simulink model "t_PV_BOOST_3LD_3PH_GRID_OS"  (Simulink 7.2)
settings: Solver=ode3  StartTime=0.0  StopTime=0.2  FixedStep=10e-6  MaxStep=1e-5  RelTol=1e-5  AbsTol=1e-5
PreLoadFcn:
  | INIT_PWM_Con
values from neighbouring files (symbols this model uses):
  I_B = INP    [INIT_PWM_Con.m]    (also in INIT_B6_2L_3Ph_IGBT_OS.m = INS; INIT_B6_3L_3Ph_IGBT_OS.m = INS; INIT_PWM_2L.m; INIT_PWM_3L.m)
  UNP = ULLP/sqrt(3)    [INIT_PWM_Con.m]    (also in INIT_B6_2L_3Ph_IGBT_OS.m; INIT_B6_3L_3Ph_IGBT_OS.m; INIT_PWM_2L.m; INIT_PWM_3L.m)
  VDC = 1200    [INIT_PWM_Con.m]    (also in INIT_B6_2L_3Ph_IGBT_OS.m = 600; INIT_B6_3L_3Ph_IGBT_OS.m = 1000; INIT_PWM_2L.m = 600; INIT_PWM_3L.m)

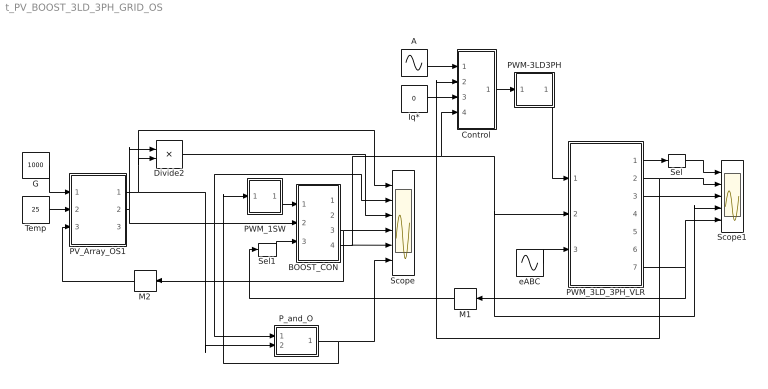
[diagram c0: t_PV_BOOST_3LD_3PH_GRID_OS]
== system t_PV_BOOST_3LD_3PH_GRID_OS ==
  A : Sin  Amplitude=.9  Frequency=2*pi*50  Phase="[0  -2*pi/3  -4*pi/3 ]"  SampleTime=0
  BOOST_CON : Subsystem  mask{L1=5e-3, IL0=100, C1=5e-3, UC0=1200, R1=1e5}
      mask prompts: L1 "Inductance L1"; IL0 "Initial Current"; C1 "Capacitance"; UC0 "Initial Voltage"; R1 "Load Resistance"
      mask help: Open Source boost Converter Input Vector u: u[0]= T1.gate u[1]= E.v u[2]= IDC.i Output Vector y: y[0]= T1.I y[1]= D1.I y[2]= L1.I y[3]= C1.V Parameter Vector p: p[0]= L1.L p[1]= L1.iL0 p[2]= C1.C p[3]= C1.vC0 p[4]= R1.r You can pause the simulation during running, change the Parameters you want and continue the Simulation
  Control : Subsystem
  Divide2 : Product  Inputs=**
  G : Constant  Value=1000  OutDataType=sfix(16)  OutScaling=2^0
  Iq* : Constant  Value=0  OutDataType=sfix(16)  OutScaling=2^0
  M1 : Memory  Orientation=left
  M2 : Memory  Orientation=left
  PV_Array_OS1 : Subsystem  mask{Isc0=5.28, Ud0=44.5, Ki=2e-3, Kv=-0.1558, n=1.0, RS=0.7, RP=400, NC=72, NMs=20, NMp=15, C=1e-4, vC0=0, RL=10000}
      mask prompts: Isc0 "Short Circuit Current at STC Isc0/Module"; Ud0 "Open Circuit Voltage at STC Ud0/Module"; Ki "Short Circuit Current Temp Coeff. Ki/Module"; Kv "Open Circuit Voltage Temp. Coeff. Kv/Module"; n "Diode Idealty Factor n"; RS "Series Resistance Rs"; RP "Parallel Resistance RP"; NC "Number Cells"; NMs "Number Series Modules"; NMp "Number Parallel Modules"; C "Load Capacitor"; vC0 "init Cap Voltage"; RL "Load Res."
      mask help: PV_Array_OS with parameters: N_Cells/Module (NC), N_Series connected Module (NMs) and N_parallel connected Module (NMp) Input Vector u: u[0]=G u[1]=T u[2]=ILd Output Vector y: y[0]=PV.I y[1]=PV.V y[2]=C.I Parameter Vector p: p[0]=Isc0 p[1]=Ud0 p[2]=Ki p[3]=Kv p[4]=n p[5]=RS p[6]=RP p[7]=NC p[8]=NMs p[9]=NMp p[10]=C p[11]=vC0 p[12]=RL You can pause the simulation during running, change the Parameters you want and continue the Simulation
  PWM-3LD3PH : Subsystem  mask(PWM-3LD3PH){FT=500, PHT=0, A=0.5, O1=0.5, O2=-0.5, DT=1e-6}
      mask prompts: FT "Frequency of Trian Sig."; PHT "Phase Angle of Trian. Sig."; A "Amplitude of Trian. Sig."; O1 "Offset of 1st Trian"; O2 "Offset of 2nd Trian."; DT "Dead Time"
      mask help: Pulse Width Modulation for 3 Phase 3 Level Neutral point clamped Converter
  PWM_1SW : Subsystem  mask(PWMtr){FS=1e3}
      mask prompts: FS "Frequency"
  PWM_3LD_3PH_VLR : Subsystem  mask(pwm_3LD_3PH_VLR_OS){RL=1e-3, LL=10e-3}
      mask prompts: RL "Load Resistance"; LL "Load Inductance"
      mask help: Open Source 3-Level NPC PWM_3PH Converter with VLR load Input Vector u: u{0:11}= gating Signals u[12]/2= VDC1, VDC2 u{13:15}= EA,EB,EC Output Vector y: y{0:2}= Va,Vb,Vc y{3:5}= Ia,Ib,Ic y[6]= Vab.V y{7:9} = T1.I,D1.I,T1.V y{10:12}= T2.I,D2.I,T2.V y[13]= D5.I y[14]= D5.V y[15]= IDC1 y[16]= IDC2 Parameter Vector p: p[0]=RL p[1]=LL You can pause the simulation during running, change the Parameters you want and continue the Simulation
  P_and_O : Subsystem  mask{DeltaD=0.0001}
      mask help: MPPT controller based on the Perturb & Observe algorithm. D output = Duty cycle of the boost converter (value between 0 and 1) DeltaD = 0.0001; Increment value used to increase/decrease the duty cycle D
  Scope : Scope  NumInputPorts=6
  Scope1 : Scope  NumInputPorts=5
  Sel : Selector  InputPortWidth=3  IndexOptions=Index vector (dialog)  Indices=[1 ]  OutputSizes=1
  Sel1 : Selector  InputPortWidth=2  IndexOptions=Index vector (dialog)  Indices=[1 ]  OutputSizes=1
  Temp : Constant  Value=25  OutDataType=sfix(16)  OutScaling=2^0
  eABC : Sin  Amplitude=UNP  Frequency=2*pi*50  Phase="[0  -2*pi/3  -4*pi/3 ]"  SampleTime=0
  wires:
  PWM_1SW/1(Out1) -> BOOST_CON/1(sw)
  P_and_O/1(D) -> PWM_1SW/1(In1), Scope/6
  PV_Array_OS1/2(PV_V) -> BOOST_CON/2(E), P_and_O/1(V), Scope/2, Divide2/1
  BOOST_CON/3(iL) -> Scope/4, M2/1
  PV_Array_OS1/1(PV_I) -> P_and_O/2(I), Divide2/2, Scope/1
  BOOST_CON/4(vC) -> Scope/5, PWM_3LD_3PH_VLR/2(vDC), Scope1/4, Control/4(UDC)
  G/1 -> PV_Array_OS1/1(G)
  Temp/1 -> PV_Array_OS1/2(Temp)
  PWM-3LD3PH/1(Out1) -> PWM_3LD_3PH_VLR/1(Sw)
  eABC/1 -> PWM_3LD_3PH_VLR/3(E_ABC)
  PWM_3LD_3PH_VLR/1(vABC) -> Sel/1
  PWM_3LD_3PH_VLR/2(iABC) -> Scope1/2, Control/2(Iwr)
  PWM_3LD_3PH_VLR/3(vAB) -> Scope1/3
  Sel/1 -> Scope1/1
  PWM_3LD_3PH_VLR/7(iDC1,iDC2) -> M1/1, Scope1/5
  M1/1 -> Sel1/1
  M2/1 -> PV_Array_OS1/3(ILd)
  A/1 -> Control/1(UNP)
  Control/1(A) -> PWM-3LD3PH/1(In1)
  Iq*/1 -> Control/3(Iq*)
  Divide2/1 -> Scope/3
  Sel1/1 -> BOOST_CON/3(IDC)

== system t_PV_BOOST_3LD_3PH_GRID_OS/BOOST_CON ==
  sw : Inport  OutDataType=sfix(16)  OutScaling=2^0
  E : Inport  Port=2  OutDataType=sfix(16)  OutScaling=2^0
  IDC : Inport  Port=3  OutDataType=sfix(16)  OutScaling=2^0
  BOOST : S-Function  FunctionName=s_boost_OS  Parameters="[L1  IL0  C1   UC0  R1]"  EnableBusSupport=off
  Mux1 : Mux  Inputs=3
  iT : Outport  OutDataType=sfix(16)  OutScaling=2^0
  iD : Outport  Port=2  OutDataType=sfix(16)  OutScaling=2^0
  iL : Outport  Port=3  OutDataType=sfix(16)  OutScaling=2^0
  vC : Outport  Port=4  OutDataType=sfix(16)  OutScaling=2^0
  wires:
  IDC/1 -> Mux1/3
  BOOST/4 -> vC/1
  BOOST/3 -> iL/1
  BOOST/2 -> iD/1
  BOOST/1 -> iT/1
  E/1 -> Mux1/2
  sw/1 -> Mux1/1
  Mux1/1 -> BOOST/1

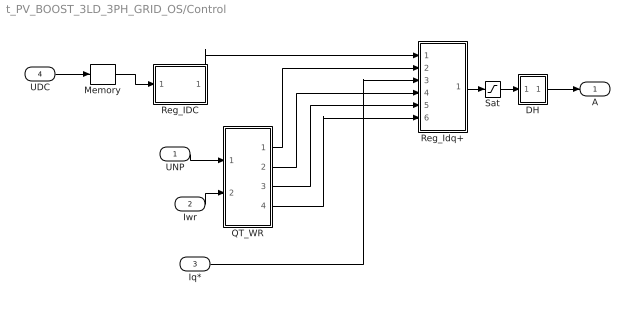
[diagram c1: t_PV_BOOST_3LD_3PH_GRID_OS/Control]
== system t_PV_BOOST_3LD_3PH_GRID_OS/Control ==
  UNP : Inport
  Iwr : Inport  Port=2
  Iq* : Inport  Port=3
  UDC : Inport  Port=4
  DH : Subsystem
  Memory : Memory
  QT_WR : Subsystem
  Reg_IDC : Subsystem
  Reg_Idq+ : Subsystem
  Sat : Saturate  UpperLimit=1  LowerLimit=-1
  A : Outport
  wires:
  QT_WR/4(Ud) -> Reg_Idq+/6(Ud)
  QT_WR/1(Id1) -> Reg_Idq+/2(Id1)
  QT_WR/2(Iq1) -> Reg_Idq+/4(Iq1)
  Iq*/1 -> Reg_Idq+/3(Iq1*)
  QT_WR/3(th1) -> Reg_Idq+/5(th)
  Iwr/1 -> QT_WR/2(I_WR)
  UNP/1 -> QT_WR/1(UNP)
  DH/1(O) -> A/1
  Reg_Idq+/1(A+) -> Sat/1
  Sat/1 -> DH/1(I)
  UDC/1 -> Memory/1
  Memory/1 -> Reg_IDC/1(UDC)
  Reg_IDC/1(Id1*) -> Reg_Idq+/1(Id1*)

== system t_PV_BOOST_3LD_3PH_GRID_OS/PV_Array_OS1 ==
  G : Inport
  Temp : Inport  Port=2
  ILd : Inport  Port=3
  Mux : Mux  Inputs=3
  t_PV_Array_OS : S-Function  FunctionName=s_PV_Array_OS  Parameters="[Isc0  Ud0  Ki  Kv  n    RS  RP NC  NMs NMp C  vC0  RL]"  EnableBusSupport=off
  PV_I : Outport
  PV_V : Outport  Port=2
  C_I : Outport  Port=3
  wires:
  Mux/1 -> t_PV_Array_OS/1
  G/1 -> Mux/1
  Temp/1 -> Mux/2
  ILd/1 -> Mux/3
  t_PV_Array_OS/1 -> PV_I/1
  t_PV_Array_OS/2 -> PV_V/1
  t_PV_Array_OS/3 -> C_I/1

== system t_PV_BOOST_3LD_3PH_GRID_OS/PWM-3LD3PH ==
  In1 : Inport  OutDataType=sfix(16)  OutScaling=2^0
  Demux1 : Demux  Outputs=3
  Mux1 : Mux  Inputs=3
  PWM-3LD1PH : Subsystem  mask(PWM-3LD_1PH){FT=FT, PHT=PHT, A=A, O1=O1, O2=O2, DT=DT}
      mask prompts: FT "Frequency of Trian Sig."; PHT "Phase Angle of Trian. Sig."; A "Amplitude of Trian. Sig."; O1 "Offset of 1st Trian"; O2 "Offset of 2nd Trian."; DT "Dead Time"
      mask help: Pulse Width Modulation for 1 Leg of 3 Level Neutral point clamped Converter
  PWM-3LD1PH1 : Subsystem  mask(PWM-3LD_1PH){FT=FT, PHT=PHT, A=A, O1=O1, O2=O2, DT=DT}
      mask prompts: FT "Frequency of Trian Sig."; PHT "Phase Angle of Trian. Sig."; A "Amplitude of Trian. Sig."; O1 "Offset of 1st Trian"; O2 "Offset of 2nd Trian."; DT "Dead Time"
      mask help: Pulse Width Modulation for 1 Leg of 3 Level Neutral point clamped Converter
  PWM-3LD1PH2 : Subsystem  mask(PWM-3LD_1PH){FT=FT, PHT=PHT, A=A, O1=O1, O2=O2, DT=DT}
      mask prompts: FT "Frequency of Trian Sig."; PHT "Phase Angle of Trian. Sig."; A "Amplitude of Trian. Sig."; O1 "Offset of 1st Trian"; O2 "Offset of 2nd Trian."; DT "Dead Time"
      mask help: Pulse Width Modulation for 1 Leg of 3 Level Neutral point clamped Converter
  Out1 : Outport
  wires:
  In1/1 -> Demux1/1
  Demux1/3 -> PWM-3LD1PH2/1(In1)
  Demux1/2 -> PWM-3LD1PH1/1(In1)
  Demux1/1 -> PWM-3LD1PH/1(In1)
  Mux1/1 -> Out1/1
  PWM-3LD1PH2/1(Out1) -> Mux1/3
  PWM-3LD1PH1/1(Out1) -> Mux1/2
  PWM-3LD1PH/1(Out1) -> Mux1/1

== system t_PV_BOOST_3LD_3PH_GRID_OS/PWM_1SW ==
  In1 : Inport  OutDataType=sfix(16)  OutScaling=2^0
  Relay : Relay  OutDataType=sfix(16)  OutScaling=2^0
  SoToG : Subsystem  mask(SoToG){T=1/FS}
      mask prompts: T "Period Time"
  Sum : Sum  Inputs=+-  OutDataType=sfix(16)  OutScaling=2^0
  Out1 : Outport  InitialOutput=0
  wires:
  Relay/1 -> Out1/1
  SoToG/1(O) -> Sum/2
  In1/1 -> Sum/1
  Sum/1 -> Relay/1

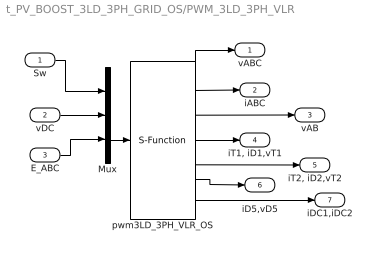
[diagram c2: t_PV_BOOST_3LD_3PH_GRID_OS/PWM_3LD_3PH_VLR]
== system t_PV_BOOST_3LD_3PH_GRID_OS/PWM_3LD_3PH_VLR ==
  Sw : Inport  OutDataType=sfix(16)  OutScaling=2^0
  vDC : Inport  Port=2  OutDataType=sfix(16)  OutScaling=2^0
  E_ABC : Inport  Port=3  OutDataType=sfix(16)  OutScaling=2^0
  Mux : Mux  Inputs="[12 1  3]"
  pwm3LD_3PH_VLR_OS : S-Function  FunctionName=s_pwm_3LD_3PH_VLR_OS  Parameters="[RL  LL]"  EnableBusSupport=off
  vABC : Outport  OutDataType=sfix(16)  OutScaling=2^0
  iABC : Outport  Port=2  OutDataType=sfix(16)  OutScaling=2^0
  vAB : Outport  Port=3  OutDataType=sfix(16)  OutScaling=2^0
  "iT1, iD1,vT1" : Outport  Port=4  OutDataType=sfix(16)  OutScaling=2^0
  "iT2, iD2,vT2" : Outport  Port=5  OutDataType=sfix(16)  OutScaling=2^0
  iD5,vD5 : Outport  Port=6  OutDataType=sfix(16)  OutScaling=2^0
  iDC1,iDC2 : Outport  Port=7  OutDataType=sfix(16)  OutScaling=2^0
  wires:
  Sw/1 -> Mux/1
  vDC/1 -> Mux/2
  Mux/1 -> pwm3LD_3PH_VLR_OS/1
  E_ABC/1 -> Mux/3
  pwm3LD_3PH_VLR_OS/1 -> vABC/1
  pwm3LD_3PH_VLR_OS/4 -> "iT1, iD1,vT1"/1
  pwm3LD_3PH_VLR_OS/2 -> iABC/1
  pwm3LD_3PH_VLR_OS/3 -> vAB/1
  pwm3LD_3PH_VLR_OS/5 -> "iT2, iD2,vT2"/1
  pwm3LD_3PH_VLR_OS/6 -> iD5,vD5/1
  pwm3LD_3PH_VLR_OS/7 -> iDC1,iDC2/1

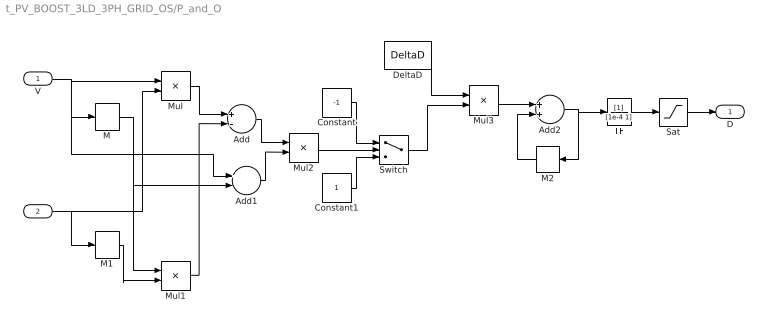
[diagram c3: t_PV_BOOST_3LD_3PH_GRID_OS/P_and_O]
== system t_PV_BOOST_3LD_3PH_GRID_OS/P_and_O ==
  V : Inport  OutDataType=sfix(16)  OutScaling=2^0
  I : Inport  Port=2  OutDataType=sfix(16)  OutScaling=2^0
  Add : Sum  Inputs=+-  OutDataType=sfix(16)  OutScaling=2^-10
  Add1 : Sum  Inputs=+-  OutDataType=sfix(16)  OutScaling=2^-10
  Add2 : Sum  OutDataType=sfix(16)  OutScaling=2^-10
  Constant : Constant  Value=-1  OutDataType=sfix(16)  OutScaling=2^0
  Constant1 : Constant  OutDataType=sfix(16)  OutScaling=2^0
  DeltaD : Constant  Value=DeltaD  OutDataType=sfix(16)  OutScaling=2^0
  M : Memory
  M1 : Memory
  M2 : Memory  Orientation=left
  Mul{,1..3} (4 alike) : Product  Inputs=**  OutDataType=sfix(16)  OutScaling=2^-10
  Sat : Saturate  UpperLimit=1  LowerLimit=0  OutDataType=sfix(16)  OutScaling=2^0
  Switch : Switch  OutDataType=sfix(16)  OutScaling=2^0
  TF : TransferFcn  Denominator=[1e-4 1]
  D : Outport  OutDataType=sfix(16)  OutScaling=2^0
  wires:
  Sat/1 -> D/1
  TF/1 -> Sat/1
  M2/1 -> Add2/2
  Add2/1 -> TF/1, M2/1
  Mul3/1 -> Add2/1
  DeltaD/1 -> Mul3/1
  Switch/1 -> Mul3/2
  Constant1/1 -> Switch/3
  Constant/1 -> Switch/1
  Mul2/1 -> Switch/2
  Add1/1 -> Mul2/2
  Add/1 -> Mul2/1
  Mul1/1 -> Add/2
  Mul/1 -> Add/1
  M1/1 -> Mul1/2
  M/1 -> Add1/2, Mul1/1
  V/1 -> Add1/1, M/1, Mul/1
  I/1 -> M1/1, Mul/2

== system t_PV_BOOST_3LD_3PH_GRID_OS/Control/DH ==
  I : Inport
  Gain : Gain  Gain=0.5
  MinMax : MinMax
  MinMax1 : MinMax  Function=max
  Sum6 : Sum  Inputs=--
  Sum7 : Sum
  O : Outport  InitialOutput=0
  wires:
  Sum7/1 -> O/1
  Gain/1 -> Sum7/2
  Sum6/1 -> Gain/1
  MinMax1/1 -> Sum6/2
  MinMax/1 -> Sum6/1
  I/1 -> Sum7/1, MinMax/1, MinMax1/1

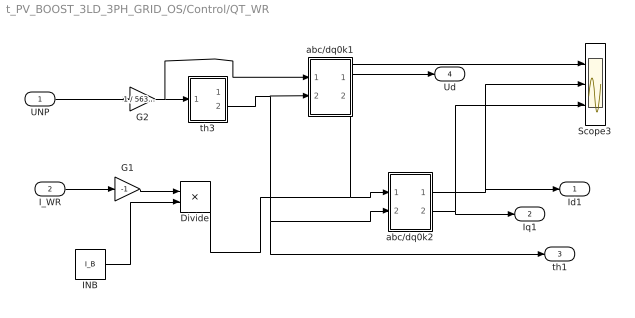
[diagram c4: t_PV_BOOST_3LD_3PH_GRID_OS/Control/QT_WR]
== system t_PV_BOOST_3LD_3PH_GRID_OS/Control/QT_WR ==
  UNP : Inport
  I_WR : Inport  Port=2
  Divide : Product  Inputs=*/  OutDataType=sfix(16)  OutScaling=2^-10
  G1 : Gain  Gain=-1
  G2 : Gain  Gain=1 / 563.39
  INB : Constant  Value=I_B  OutDataType=sfix(16)  OutScaling=2^0
  Scope3 : Scope  NumInputPorts=3
  abc/dq0k1 : Subsystem
  abc/dq0k2 : Subsystem
  th3 : Subsystem
  Id1 : Outport
  Iq1 : Outport  Port=2
  th1 : Outport  Port=3
  Ud : Outport  Port=4
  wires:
  INB/1 -> Divide/2
  G1/1 -> Divide/1
  Divide/1 -> Scope3/1, abc/dq0k2/1(a)
  UNP/1 -> G2/1
  abc/dq0k1/1(dk) -> Ud/1
  abc/dq0k2/2(qk) -> Scope3/3, Iq1/1
  abc/dq0k2/1(dk) -> Scope3/2, Id1/1
  G2/1 -> abc/dq0k1/1(a), th3/1(abc)
  I_WR/1 -> G1/1
  th3/2(th) -> abc/dq0k2/2(th), th1/1, abc/dq0k1/2(th)

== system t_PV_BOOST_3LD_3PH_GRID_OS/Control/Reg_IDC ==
  UDC : Inport
  Add : Sum
  G4 : Gain  Gain=1/VDC
  PIC1 : Subsystem  mask(PI-controller){Kp=20, Ki=10, Kd=0, lim=10, Ts=-10}
      mask prompts: Kp "Proportional gain (Kp)"; Ki "Integral gain (Ki)"; Kd "Diff. gain (Kd)"; lim "Output limit"; Ts "Sampling time (s)"
      mask help: Proportional-Integral Controller
  Sat : Saturate  UpperLimit=2  LowerLimit=-2
  UC_Reg : Scope  NumInputPorts=3
  UDC* : Constant  Value=1.0
  Id1* : Outport
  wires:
  UDC/1 -> G4/1
  UDC*/1 -> PIC1/1(c*)
  G4/1 -> PIC1/2(c), UC_Reg/3
  PIC1/1(e*) -> UC_Reg/2, Add/2
  Add/1 -> Sat/1
  Sat/1 -> Id1*/1, UC_Reg/1

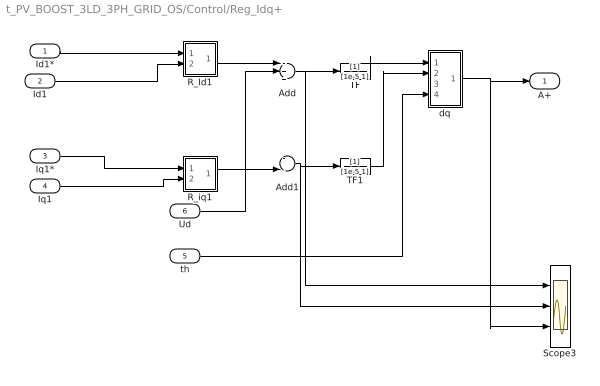
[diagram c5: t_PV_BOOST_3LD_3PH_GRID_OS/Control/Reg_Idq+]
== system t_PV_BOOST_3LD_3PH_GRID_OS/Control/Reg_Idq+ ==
  Id1* : Inport
  Id1 : Inport  Port=2
  Iq1* : Inport  Port=3
  Iq1 : Inport  Port=4
  th : Inport  Port=5
  Ud : Inport  Port=6
  Add : Sum  Inputs=-++
  Add1 : Sum  Inputs=--
  R_Id1 : Subsystem  mask(PI-controller){Kp=1, Ki=100, lim=2, Ts=-1}
      mask prompts: Kp "Proportional gain (Kp)"; Ki "Integral gain (Ki)"; lim "Output limit"; Ts "Sampling time (s)"
      mask help: Proportional-Integral Controller
  R_iq1 : Subsystem  mask(PI-controller){Kp=1, Ki=100, lim=2, Ts=-2}
      mask prompts: Kp "Proportional gain (Kp)"; Ki "Integral gain (Ki)"; lim "Output limit"; Ts "Sampling time (s)"
      mask help: Proportional-Integral Controller
  Scope3 : Scope  NumInputPorts=3
  TF : TransferFcn  Denominator=[1e-5 1]
  TF1 : TransferFcn  Denominator=[1e-5 1]
  dq : Subsystem
  A+ : Outport
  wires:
  Ud/1 -> Add/2
  TF1/1 -> dq/2(qk)
  TF/1 -> dq/1(dk)
  Add1/1 -> Scope3/2, TF1/1
  Add/1 -> Scope3/1, TF/1
  R_iq1/1(e*) -> Add1/2
  R_Id1/1(e*) -> Add/1
  th/1 -> dq/4(th)
  dq/1(a) -> Scope3/3, A+/1
  Id1*/1 -> R_Id1/1(c*)
  Id1/1 -> R_Id1/2(c)
  Iq1*/1 -> R_iq1/1(c*)
  Iq1/1 -> R_iq1/2(c)

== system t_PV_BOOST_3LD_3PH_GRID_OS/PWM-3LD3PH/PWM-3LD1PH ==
  In1 : Inport  OutDataType=sfix(16)  OutScaling=2^0
  Mux : Mux
  SS : Subsystem
  SS1 : Subsystem
  Out1 : Outport
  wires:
  In1/1 -> SS1/1(I1), SS/1(I1)
  SS1/1(O1) -> Mux/2
  SS/2(O2) -> Mux/3
  Mux/1 -> Out1/1
  SS/1(O1) -> Mux/1
  SS1/2(O2) -> Mux/4

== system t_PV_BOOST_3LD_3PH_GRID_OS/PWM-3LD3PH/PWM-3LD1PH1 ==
  In1 : Inport  OutDataType=sfix(16)  OutScaling=2^0
  Mux : Mux
  SS : Subsystem
  SS1 : Subsystem
  Out1 : Outport
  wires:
  SS1/2(O2) -> Mux/4
  SS/1(O1) -> Mux/1
  Mux/1 -> Out1/1
  SS/2(O2) -> Mux/3
  SS1/1(O1) -> Mux/2
  In1/1 -> SS/1(I1), SS1/1(I1)

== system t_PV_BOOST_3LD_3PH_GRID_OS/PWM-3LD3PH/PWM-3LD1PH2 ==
  In1 : Inport  OutDataType=sfix(16)  OutScaling=2^0
  Mux : Mux
  SS : Subsystem
  SS1 : Subsystem
  Out1 : Outport
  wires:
  In1/1 -> SS1/1(I1), SS/1(I1)
  SS1/1(O1) -> Mux/2
  SS/2(O2) -> Mux/3
  Mux/1 -> Out1/1
  SS/1(O1) -> Mux/1
  SS1/2(O2) -> Mux/4

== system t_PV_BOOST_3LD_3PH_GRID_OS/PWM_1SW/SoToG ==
  Clock : Clock
  P : Product  OutDataType=sfix(16)  OutScaling=2^0
  T1 : Constant  Value=T  OutDataType=sfix(16)  OutScaling=2^0
  T2 : Constant  Value=1/T  OutDataType=sfix(16)  OutScaling=2^0
  mod : Math  Operator=mod
  O : Outport
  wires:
  P/1 -> O/1
  mod/1 -> P/1
  T2/1 -> P/2
  T1/1 -> mod/2
  Clock/1 -> mod/1

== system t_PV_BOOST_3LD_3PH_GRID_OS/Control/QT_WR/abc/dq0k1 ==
  a : Inport
  th : Inport  Port=2
  Demux : Demux  Outputs=3
  Fcn : Fcn  Expr=u(1)*cos(u(3)) + u(2)*sin(u(3))
  Fcn1 : Fcn  Expr=-u(1)*sin(u(3)) + u(2)*cos(u(3))
  K : Gain  Gain="2/3*[1   -.5   -.5;  0   sqrt(3)/2   -sqrt(3)/2;  .5    .5    .5]"  Multiplication=Matrix(K*u)
  Mux1 : Mux  Inputs=3
  dk : Outport
  qk : Outport  Port=2
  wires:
  K/1 -> Demux/1
  a/1 -> K/1
  Mux1/1 -> Fcn1/1, Fcn/1
  Fcn/1 -> dk/1
  Fcn1/1 -> qk/1
  th/1 -> Mux1/3
  Demux/1 -> Mux1/1
  Demux/2 -> Mux1/2

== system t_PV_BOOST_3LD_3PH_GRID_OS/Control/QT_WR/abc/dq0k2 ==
  a : Inport
  th : Inport  Port=2
  Demux : Demux  Outputs=3
  Fcn : Fcn  Expr=u(1)*cos(u(3)) + u(2)*sin(u(3))
  Fcn1 : Fcn  Expr=-u(1)*sin(u(3)) + u(2)*cos(u(3))
  K : Gain  Gain="2/3*[1   -.5   -.5;  0   sqrt(3)/2   -sqrt(3)/2;  .5    .5    .5]"  Multiplication=Matrix(K*u)
  Mux1 : Mux  Inputs=3
  dk : Outport
  qk : Outport  Port=2
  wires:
  Demux/2 -> Mux1/2
  Demux/1 -> Mux1/1
  th/1 -> Mux1/3
  Fcn1/1 -> qk/1
  Fcn/1 -> dk/1
  Mux1/1 -> Fcn/1, Fcn1/1
  a/1 -> K/1
  K/1 -> Demux/1

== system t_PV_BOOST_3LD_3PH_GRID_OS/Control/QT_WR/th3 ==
  abc : Inport
  C : ComplexToMagnitudeAngle
  Demux : Demux  Outputs=3
  K : Gain  Gain="2/3*[1   -.5   -.5;  0   sqrt(3)/2   -sqrt(3)/2;  .5    .5    .5]"  Multiplication=Matrix(K*u)
  R : RealImagToComplex
  |u| : Outport
  th : Outport  Port=2
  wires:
  C/1 -> |u|/1
  K/1 -> Demux/1
  abc/1 -> K/1
  Demux/1 -> R/1
  Demux/2 -> R/2
  R/1 -> C/1
  C/2 -> th/1

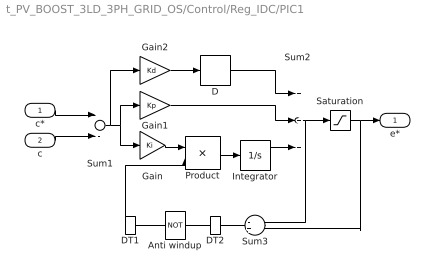
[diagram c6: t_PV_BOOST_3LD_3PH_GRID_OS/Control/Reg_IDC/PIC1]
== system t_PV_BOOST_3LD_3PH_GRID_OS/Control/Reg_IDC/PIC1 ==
  c* : Inport
  c : Inport  Port=2
  Anti windup : Logic  Operator=NOT
  D : Derivative
  DT1 : DataTypeConversion
  DT2 : DataTypeConversion
  Gain : Gain  Gain=Ki
  Gain1 : Gain  Gain=Kp
  Gain2 : Gain  Gain=Kd
  Integrator : Integrator  UpperSaturationLimit=lim  LowerSaturationLimit=-lim
  Product : Product
  Saturation : Saturate  UpperLimit=lim  LowerLimit=-lim
  Sum1 : Sum  Inputs=+-
  Sum2 : Sum  Inputs=+++
  Sum3 : Sum  Inputs=-+
  e* : Outport  InitialOutput=0
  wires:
  Sum3/1 -> DT2/1
  DT2/1 -> Anti windup/1
  Product/1 -> Integrator/1
  Gain/1 -> Product/1
  DT1/1 -> Product/2
  Anti windup/1 -> DT1/1
  Gain1/1 -> Sum2/2
  Sum1/1 -> Gain/1, Gain1/1, Gain2/1
  Sum2/1 -> Sum3/1, Saturation/1
  Saturation/1 -> Sum3/2, e*/1
  c/1 -> Sum1/2
  c*/1 -> Sum1/1
  Integrator/1 -> Sum2/3
  Gain2/1 -> D/1
  D/1 -> Sum2/1

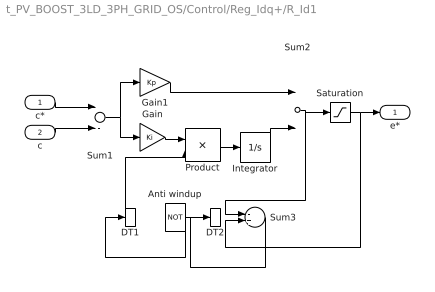
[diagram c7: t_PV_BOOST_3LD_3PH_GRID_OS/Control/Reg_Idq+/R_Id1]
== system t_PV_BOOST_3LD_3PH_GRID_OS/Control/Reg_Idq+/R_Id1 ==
  c* : Inport
  c : Inport  Port=2
  Anti windup : Logic  Operator=NOT
  DT1 : DataTypeConversion
  DT2 : DataTypeConversion
  Gain : Gain  Gain=Ki
  Gain1 : Gain  Gain=Kp
  Integrator : Integrator  UpperSaturationLimit=lim  LowerSaturationLimit=-lim
  Product : Product
  Saturation : Saturate  UpperLimit=lim  LowerLimit=-lim
  Sum1 : Sum  Inputs=+-
  Sum2 : Sum
  Sum3 : Sum  Inputs=-+
  e* : Outport  InitialOutput=0
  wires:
  Sum3/1 -> DT2/1
  DT2/1 -> Anti windup/1
  Product/1 -> Integrator/1
  Gain/1 -> Product/1
  DT1/1 -> Product/2
  Anti windup/1 -> DT1/1
  Gain1/1 -> Sum2/1
  Sum1/1 -> Gain/1, Gain1/1
  Sum2/1 -> Sum3/1, Saturation/1
  Saturation/1 -> Sum3/2, e*/1
  c/1 -> Sum1/2
  c*/1 -> Sum1/1
  Integrator/1 -> Sum2/2

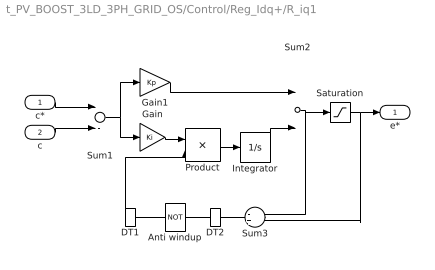
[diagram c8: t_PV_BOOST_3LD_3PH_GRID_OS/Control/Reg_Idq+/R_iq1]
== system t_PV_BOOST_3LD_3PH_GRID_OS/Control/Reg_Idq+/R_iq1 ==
  c* : Inport
  c : Inport  Port=2
  Anti windup : Logic  Operator=NOT
  DT1 : DataTypeConversion
  DT2 : DataTypeConversion
  Gain : Gain  Gain=Ki
  Gain1 : Gain  Gain=Kp
  Integrator : Integrator  UpperSaturationLimit=lim  LowerSaturationLimit=-lim
  Product : Product
  Saturation : Saturate  UpperLimit=lim  LowerLimit=-lim
  Sum1 : Sum  Inputs=+-
  Sum2 : Sum
  Sum3 : Sum  Inputs=-+
  e* : Outport  InitialOutput=0
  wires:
  Integrator/1 -> Sum2/2
  c*/1 -> Sum1/1
  c/1 -> Sum1/2
  Saturation/1 -> e*/1, Sum3/2
  Sum2/1 -> Saturation/1, Sum3/1
  Sum1/1 -> Gain1/1, Gain/1
  Gain1/1 -> Sum2/1
  Anti windup/1 -> DT1/1
  DT1/1 -> Product/2
  Gain/1 -> Product/1
  Product/1 -> Integrator/1
  DT2/1 -> Anti windup/1
  Sum3/1 -> DT2/1

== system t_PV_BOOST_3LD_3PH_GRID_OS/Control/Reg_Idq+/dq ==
  dk : Inport
  qk : Inport  Port=2
  0k : Inport  Port=3
  th : Inport  Port=4
  Fcn : Fcn  Expr=u(1)*cos(u(3)) - u(2)*sin(u(3))
  Fcn1 : Fcn  Expr=u(1)*sin(u(3)) + u(2)*cos(u(3))
  K : Gain  Gain="[1   0  1 ;  -.5   sqrt(3)/2    1 ;  -.5    -sqrt(3)/2    1]"  Multiplication=Matrix(K*u)
  Mux : Mux  Inputs=3
  Mux1 : Mux  Inputs=3
  a : Outport
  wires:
  dk/1 -> Mux/1
  qk/1 -> Mux/2
  Mux/1 -> Fcn/1, Fcn1/1
  K/1 -> a/1
  Mux1/1 -> K/1
  Fcn/1 -> Mux1/1
  Fcn1/1 -> Mux1/2
  th/1 -> Mux/3
  0k/1 -> Mux1/3

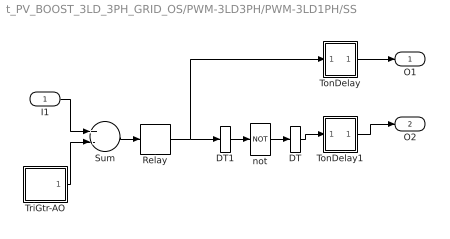
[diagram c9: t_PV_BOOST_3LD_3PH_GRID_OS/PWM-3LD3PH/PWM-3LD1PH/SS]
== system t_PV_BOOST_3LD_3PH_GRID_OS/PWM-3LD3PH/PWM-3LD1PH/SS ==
  I1 : Inport  OutDataType=sfix(16)  OutScaling=2^0
  DT : DataTypeConversion
  DT1 : DataTypeConversion
  Relay : Relay  OutDataType=sfix(16)  OutScaling=2^0
  Sum : Sum  Inputs=+-  OutDataType=sfix(16)  OutScaling=2^0
  TonDelay : Subsystem  mask(TonDelay){DT=DT}
      mask prompts: DT "Dead Time"
      mask help: Turn on dead time to protect against short circuit of the converter leg
  TonDelay1 : Subsystem  mask(TonDelay){DT=DT}
      mask prompts: DT "Dead Time"
      mask help: Turn on dead time to protect against short circuit of the converter leg
  TriGtr-AO : Subsystem  mask(TriGtr-AO){A=A, O=O1, T=1/FT, Td=PHT/FT/180}
      mask prompts: A "Amplitude"; O "Offset"; T "Period Time"; Td "Time Delay"
      mask help: Triangular Wave Generator with variable time delay, variable amplitude and offset
  not : Logic  Operator=NOT  Inputs=1
  O1 : Outport  InitialOutput=0
  O2 : Outport  Port=2  InitialOutput=0
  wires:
  TonDelay/1(s1d) -> O1/1
  Relay/1 -> TonDelay/1(s1), DT1/1
  TonDelay1/1(s1d) -> O2/1
  not/1 -> DT/1
  Sum/1 -> Relay/1
  TriGtr-AO/1(Out1) -> Sum/2
  I1/1 -> Sum/1
  DT/1 -> TonDelay1/1(s1)
  DT1/1 -> not/1

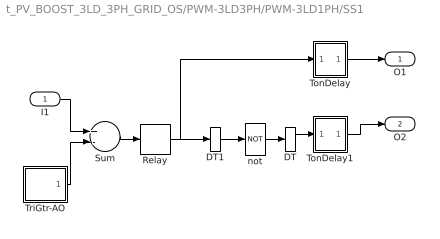
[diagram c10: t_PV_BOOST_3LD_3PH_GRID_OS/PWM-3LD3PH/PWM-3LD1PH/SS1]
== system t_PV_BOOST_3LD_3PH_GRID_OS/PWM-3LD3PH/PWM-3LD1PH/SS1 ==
  I1 : Inport  OutDataType=sfix(16)  OutScaling=2^0
  DT : DataTypeConversion
  DT1 : DataTypeConversion
  Relay : Relay  OutDataType=sfix(16)  OutScaling=2^0
  Sum : Sum  Inputs=+-  OutDataType=sfix(16)  OutScaling=2^0
  TonDelay : Subsystem  mask(TonDelay){DT=DT}
      mask prompts: DT "Dead Time"
      mask help: Turn on dead time to protect against short circuit of the converter leg
  TonDelay1 : Subsystem  mask(TonDelay){DT=DT}
      mask prompts: DT "Dead Time"
      mask help: Turn on dead time to protect against short circuit of the converter leg
  TriGtr-AO : Subsystem  mask(TriGtr-AO){A=A, O=O2, T=1/FT, Td=PHT/FT/180}
      mask prompts: A "Amplitude"; O "Offset"; T "Period Time"; Td "Time Delay"
      mask help: Triangular Wave Generator with variable time delay, variable amplitude and offset
  not : Logic  Operator=NOT  Inputs=1
  O1 : Outport  InitialOutput=0
  O2 : Outport  Port=2  InitialOutput=0
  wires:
  TonDelay/1(s1d) -> O1/1
  Relay/1 -> TonDelay/1(s1), DT1/1
  TonDelay1/1(s1d) -> O2/1
  not/1 -> DT/1
  Sum/1 -> Relay/1
  TriGtr-AO/1(Out1) -> Sum/2
  I1/1 -> Sum/1
  DT/1 -> TonDelay1/1(s1)
  DT1/1 -> not/1

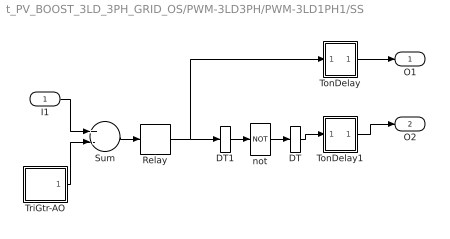
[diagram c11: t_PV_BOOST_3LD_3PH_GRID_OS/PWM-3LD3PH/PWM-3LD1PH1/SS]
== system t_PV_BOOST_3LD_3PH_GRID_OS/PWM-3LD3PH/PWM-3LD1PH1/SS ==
  I1 : Inport  OutDataType=sfix(16)  OutScaling=2^0
  DT : DataTypeConversion
  DT1 : DataTypeConversion
  Relay : Relay  OutDataType=sfix(16)  OutScaling=2^0
  Sum : Sum  Inputs=+-  OutDataType=sfix(16)  OutScaling=2^0
  TonDelay : Subsystem  mask(TonDelay){DT=DT}
      mask prompts: DT "Dead Time"
      mask help: Turn on dead time to protect against short circuit of the converter leg
  TonDelay1 : Subsystem  mask(TonDelay){DT=DT}
      mask prompts: DT "Dead Time"
      mask help: Turn on dead time to protect against short circuit of the converter leg
  TriGtr-AO : Subsystem  mask(TriGtr-AO){A=A, O=O1, T=1/FT, Td=PHT/FT/180}
      mask prompts: A "Amplitude"; O "Offset"; T "Period Time"; Td "Time Delay"
      mask help: Triangular Wave Generator with variable time delay, variable amplitude and offset
  not : Logic  Operator=NOT  Inputs=1
  O1 : Outport  InitialOutput=0
  O2 : Outport  Port=2  InitialOutput=0
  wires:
  DT1/1 -> not/1
  DT/1 -> TonDelay1/1(s1)
  I1/1 -> Sum/1
  TriGtr-AO/1(Out1) -> Sum/2
  Sum/1 -> Relay/1
  not/1 -> DT/1
  TonDelay1/1(s1d) -> O2/1
  Relay/1 -> DT1/1, TonDelay/1(s1)
  TonDelay/1(s1d) -> O1/1

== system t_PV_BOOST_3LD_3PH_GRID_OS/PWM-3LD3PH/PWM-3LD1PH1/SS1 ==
  I1 : Inport  OutDataType=sfix(16)  OutScaling=2^0
  DT : DataTypeConversion
  DT1 : DataTypeConversion
  Relay : Relay  OutDataType=sfix(16)  OutScaling=2^0
  Sum : Sum  Inputs=+-  OutDataType=sfix(16)  OutScaling=2^0
  TonDelay : Subsystem  mask(TonDelay){DT=DT}
      mask prompts: DT "Dead Time"
      mask help: Turn on dead time to protect against short circuit of the converter leg
  TonDelay1 : Subsystem  mask(TonDelay){DT=DT}
      mask prompts: DT "Dead Time"
      mask help: Turn on dead time to protect against short circuit of the converter leg
  TriGtr-AO : Subsystem  mask(TriGtr-AO){A=A, O=O2, T=1/FT, Td=PHT/FT/180}
      mask prompts: A "Amplitude"; O "Offset"; T "Period Time"; Td "Time Delay"
      mask help: Triangular Wave Generator with variable time delay, variable amplitude and offset
  not : Logic  Operator=NOT  Inputs=1
  O1 : Outport  InitialOutput=0
  O2 : Outport  Port=2  InitialOutput=0
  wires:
  DT1/1 -> not/1
  DT/1 -> TonDelay1/1(s1)
  I1/1 -> Sum/1
  TriGtr-AO/1(Out1) -> Sum/2
  Sum/1 -> Relay/1
  not/1 -> DT/1
  TonDelay1/1(s1d) -> O2/1
  Relay/1 -> DT1/1, TonDelay/1(s1)
  TonDelay/1(s1d) -> O1/1

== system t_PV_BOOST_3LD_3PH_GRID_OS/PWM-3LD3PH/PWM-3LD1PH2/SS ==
  I1 : Inport  OutDataType=sfix(16)  OutScaling=2^0
  DT : DataTypeConversion
  DT1 : DataTypeConversion
  Relay : Relay  OutDataType=sfix(16)  OutScaling=2^0
  Sum : Sum  Inputs=+-  OutDataType=sfix(16)  OutScaling=2^0
  TonDelay : Subsystem  mask(TonDelay){DT=DT}
      mask prompts: DT "Dead Time"
      mask help: Turn on dead time to protect against short circuit of the converter leg
  TonDelay1 : Subsystem  mask(TonDelay){DT=DT}
      mask prompts: DT "Dead Time"
      mask help: Turn on dead time to protect against short circuit of the converter leg
  TriGtr-AO : Subsystem  mask(TriGtr-AO){A=A, O=O1, T=1/FT, Td=PHT/FT/180}
      mask prompts: A "Amplitude"; O "Offset"; T "Period Time"; Td "Time Delay"
      mask help: Triangular Wave Generator with variable time delay, variable amplitude and offset
  not : Logic  Operator=NOT  Inputs=1
  O1 : Outport  InitialOutput=0
  O2 : Outport  Port=2  InitialOutput=0
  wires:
  TonDelay/1(s1d) -> O1/1
  Relay/1 -> TonDelay/1(s1), DT1/1
  TonDelay1/1(s1d) -> O2/1
  not/1 -> DT/1
  Sum/1 -> Relay/1
  TriGtr-AO/1(Out1) -> Sum/2
  I1/1 -> Sum/1
  DT/1 -> TonDelay1/1(s1)
  DT1/1 -> not/1

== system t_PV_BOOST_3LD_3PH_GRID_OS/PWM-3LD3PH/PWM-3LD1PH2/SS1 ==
  I1 : Inport  OutDataType=sfix(16)  OutScaling=2^0
  DT : DataTypeConversion
  DT1 : DataTypeConversion
  Relay : Relay  OutDataType=sfix(16)  OutScaling=2^0
  Sum : Sum  Inputs=+-  OutDataType=sfix(16)  OutScaling=2^0
  TonDelay : Subsystem  mask(TonDelay){DT=DT}
      mask prompts: DT "Dead Time"
      mask help: Turn on dead time to protect against short circuit of the converter leg
  TonDelay1 : Subsystem  mask(TonDelay){DT=DT}
      mask prompts: DT "Dead Time"
      mask help: Turn on dead time to protect against short circuit of the converter leg
  TriGtr-AO : Subsystem  mask(TriGtr-AO){A=A, O=O2, T=1/FT, Td=PHT/FT/180}
      mask prompts: A "Amplitude"; O "Offset"; T "Period Time"; Td "Time Delay"
      mask help: Triangular Wave Generator with variable time delay, variable amplitude and offset
  not : Logic  Operator=NOT  Inputs=1
  O1 : Outport  InitialOutput=0
  O2 : Outport  Port=2  InitialOutput=0
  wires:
  TonDelay/1(s1d) -> O1/1
  Relay/1 -> TonDelay/1(s1), DT1/1
  TonDelay1/1(s1d) -> O2/1
  not/1 -> DT/1
  Sum/1 -> Relay/1
  TriGtr-AO/1(Out1) -> Sum/2
  I1/1 -> Sum/1
  DT/1 -> TonDelay1/1(s1)
  DT1/1 -> not/1

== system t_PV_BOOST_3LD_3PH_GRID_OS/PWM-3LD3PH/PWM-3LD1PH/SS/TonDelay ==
  s1 : Inport  Orientation=down  OutDataType=sfix(16)  OutScaling=2^0
  Int : Integrator  ExternalReset=falling
  Rel1 : Relay  OnSwitchValue=DT  OutDataType=sfix(16)  OutScaling=2^0
  s1d : Outport  InitialOutput=0
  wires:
  Rel1/1 -> s1d/1
  s1/1 -> Int/1, Int/2
  Int/1 -> Rel1/1

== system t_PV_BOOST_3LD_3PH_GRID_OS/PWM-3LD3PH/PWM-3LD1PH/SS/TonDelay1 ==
  s1 : Inport  Orientation=down  OutDataType=sfix(16)  OutScaling=2^0
  Int : Integrator  ExternalReset=falling
  Rel1 : Relay  OnSwitchValue=DT  OutDataType=sfix(16)  OutScaling=2^0
  s1d : Outport  InitialOutput=0
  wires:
  Rel1/1 -> s1d/1
  s1/1 -> Int/1, Int/2
  Int/1 -> Rel1/1

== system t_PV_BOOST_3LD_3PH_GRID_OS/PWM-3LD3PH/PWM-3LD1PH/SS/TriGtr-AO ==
  Ampl. : Gain  Gain=A  ParameterDataType=sfix(16)  ParameterScaling=2^0  OutDataType=sfix(16)  OutScaling=2^0
  Offset : Constant  Value=O  OutDataType=sfix(16)  OutScaling=2^0
  Sum : Sum  OutDataType=sfix(16)  OutScaling=2^0
  TriGtr1 : Subsystem  mask(TriGtr){T=T, Td=Td}
      mask prompts: T "Period Time"; Td "Time Delay"
      mask help: Triangular Wave Generator with variable time delay
  Out1 : Outport
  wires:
  Sum/1 -> Out1/1
  Ampl./1 -> Sum/1
  TriGtr1/1(O) -> Ampl./1
  Offset/1 -> Sum/2

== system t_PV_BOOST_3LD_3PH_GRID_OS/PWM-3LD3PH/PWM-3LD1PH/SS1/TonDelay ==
  s1 : Inport  Orientation=down  OutDataType=sfix(16)  OutScaling=2^0
  Int : Integrator  ExternalReset=falling
  Rel1 : Relay  OnSwitchValue=DT  OutDataType=sfix(16)  OutScaling=2^0
  s1d : Outport  InitialOutput=0
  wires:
  Rel1/1 -> s1d/1
  s1/1 -> Int/1, Int/2
  Int/1 -> Rel1/1

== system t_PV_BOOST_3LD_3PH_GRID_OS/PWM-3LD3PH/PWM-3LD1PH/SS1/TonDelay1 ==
  s1 : Inport  Orientation=down  OutDataType=sfix(16)  OutScaling=2^0
  Int : Integrator  ExternalReset=falling
  Rel1 : Relay  OnSwitchValue=DT  OutDataType=sfix(16)  OutScaling=2^0
  s1d : Outport  InitialOutput=0
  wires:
  Rel1/1 -> s1d/1
  s1/1 -> Int/1, Int/2
  Int/1 -> Rel1/1

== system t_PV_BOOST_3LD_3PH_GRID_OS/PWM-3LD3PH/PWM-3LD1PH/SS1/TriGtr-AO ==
  Ampl. : Gain  Gain=A  ParameterDataType=sfix(16)  ParameterScaling=2^0  OutDataType=sfix(16)  OutScaling=2^0
  Offset : Constant  Value=O  OutDataType=sfix(16)  OutScaling=2^0
  Sum : Sum  OutDataType=sfix(16)  OutScaling=2^0
  TriGtr1 : Subsystem  mask(TriGtr){T=T, Td=Td}
      mask prompts: T "Period Time"; Td "Time Delay"
      mask help: Triangular Wave Generator with variable time delay
  Out1 : Outport
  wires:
  Offset/1 -> Sum/2
  TriGtr1/1(O) -> Ampl./1
  Ampl./1 -> Sum/1
  Sum/1 -> Out1/1

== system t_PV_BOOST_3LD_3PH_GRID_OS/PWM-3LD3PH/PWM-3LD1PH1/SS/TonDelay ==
  s1 : Inport  Orientation=down  OutDataType=sfix(16)  OutScaling=2^0
  Int : Integrator  ExternalReset=falling
  Rel1 : Relay  OnSwitchValue=DT  OutDataType=sfix(16)  OutScaling=2^0
  s1d : Outport  InitialOutput=0
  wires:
  Int/1 -> Rel1/1
  s1/1 -> Int/2, Int/1
  Rel1/1 -> s1d/1

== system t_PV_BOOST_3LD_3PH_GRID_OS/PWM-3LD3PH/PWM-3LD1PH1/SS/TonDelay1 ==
  s1 : Inport  Orientation=down  OutDataType=sfix(16)  OutScaling=2^0
  Int : Integrator  ExternalReset=falling
  Rel1 : Relay  OnSwitchValue=DT  OutDataType=sfix(16)  OutScaling=2^0
  s1d : Outport  InitialOutput=0
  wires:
  Int/1 -> Rel1/1
  s1/1 -> Int/2, Int/1
  Rel1/1 -> s1d/1

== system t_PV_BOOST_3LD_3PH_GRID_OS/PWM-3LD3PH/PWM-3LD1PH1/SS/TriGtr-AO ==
  Ampl. : Gain  Gain=A  ParameterDataType=sfix(16)  ParameterScaling=2^0  OutDataType=sfix(16)  OutScaling=2^0
  Offset : Constant  Value=O  OutDataType=sfix(16)  OutScaling=2^0
  Sum : Sum  OutDataType=sfix(16)  OutScaling=2^0
  TriGtr1 : Subsystem  mask(TriGtr){T=T, Td=Td}
      mask prompts: T "Period Time"; Td "Time Delay"
      mask help: Triangular Wave Generator with variable time delay
  Out1 : Outport
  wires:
  Offset/1 -> Sum/2
  TriGtr1/1(O) -> Ampl./1
  Ampl./1 -> Sum/1
  Sum/1 -> Out1/1

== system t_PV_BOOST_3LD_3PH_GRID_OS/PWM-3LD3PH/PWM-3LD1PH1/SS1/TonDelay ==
  s1 : Inport  Orientation=down  OutDataType=sfix(16)  OutScaling=2^0
  Int : Integrator  ExternalReset=falling
  Rel1 : Relay  OnSwitchValue=DT  OutDataType=sfix(16)  OutScaling=2^0
  s1d : Outport  InitialOutput=0
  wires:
  Int/1 -> Rel1/1
  s1/1 -> Int/2, Int/1
  Rel1/1 -> s1d/1

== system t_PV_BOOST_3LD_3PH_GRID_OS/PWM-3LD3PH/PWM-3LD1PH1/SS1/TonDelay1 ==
  s1 : Inport  Orientation=down  OutDataType=sfix(16)  OutScaling=2^0
  Int : Integrator  ExternalReset=falling
  Rel1 : Relay  OnSwitchValue=DT  OutDataType=sfix(16)  OutScaling=2^0
  s1d : Outport  InitialOutput=0
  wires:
  Int/1 -> Rel1/1
  s1/1 -> Int/2, Int/1
  Rel1/1 -> s1d/1

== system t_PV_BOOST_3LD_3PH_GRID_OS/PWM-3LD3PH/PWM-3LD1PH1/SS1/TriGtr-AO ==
  Ampl. : Gain  Gain=A  ParameterDataType=sfix(16)  ParameterScaling=2^0  OutDataType=sfix(16)  OutScaling=2^0
  Offset : Constant  Value=O  OutDataType=sfix(16)  OutScaling=2^0
  Sum : Sum  OutDataType=sfix(16)  OutScaling=2^0
  TriGtr1 : Subsystem  mask(TriGtr){T=T, Td=Td}
      mask prompts: T "Period Time"; Td "Time Delay"
      mask help: Triangular Wave Generator with variable time delay
  Out1 : Outport
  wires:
  Sum/1 -> Out1/1
  Ampl./1 -> Sum/1
  TriGtr1/1(O) -> Ampl./1
  Offset/1 -> Sum/2

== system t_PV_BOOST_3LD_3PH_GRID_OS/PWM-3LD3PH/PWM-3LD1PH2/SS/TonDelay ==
  s1 : Inport  Orientation=down  OutDataType=sfix(16)  OutScaling=2^0
  Int : Integrator  ExternalReset=falling
  Rel1 : Relay  OnSwitchValue=DT  OutDataType=sfix(16)  OutScaling=2^0
  s1d : Outport  InitialOutput=0
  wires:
  Rel1/1 -> s1d/1
  s1/1 -> Int/1, Int/2
  Int/1 -> Rel1/1

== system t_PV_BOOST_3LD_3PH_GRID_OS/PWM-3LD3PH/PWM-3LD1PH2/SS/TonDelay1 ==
  s1 : Inport  Orientation=down  OutDataType=sfix(16)  OutScaling=2^0
  Int : Integrator  ExternalReset=falling
  Rel1 : Relay  OnSwitchValue=DT  OutDataType=sfix(16)  OutScaling=2^0
  s1d : Outport  InitialOutput=0
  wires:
  Rel1/1 -> s1d/1
  s1/1 -> Int/1, Int/2
  Int/1 -> Rel1/1

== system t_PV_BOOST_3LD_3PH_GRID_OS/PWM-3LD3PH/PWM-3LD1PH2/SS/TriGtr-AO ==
  Ampl. : Gain  Gain=A  ParameterDataType=sfix(16)  ParameterScaling=2^0  OutDataType=sfix(16)  OutScaling=2^0
  Offset : Constant  Value=O  OutDataType=sfix(16)  OutScaling=2^0
  Sum : Sum  OutDataType=sfix(16)  OutScaling=2^0
  TriGtr1 : Subsystem  mask(TriGtr){T=T, Td=Td}
      mask prompts: T "Period Time"; Td "Time Delay"
      mask help: Triangular Wave Generator with variable time delay
  Out1 : Outport
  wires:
  Sum/1 -> Out1/1
  Ampl./1 -> Sum/1
  TriGtr1/1(O) -> Ampl./1
  Offset/1 -> Sum/2

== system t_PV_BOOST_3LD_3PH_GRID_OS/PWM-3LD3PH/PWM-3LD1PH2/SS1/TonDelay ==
  s1 : Inport  Orientation=down  OutDataType=sfix(16)  OutScaling=2^0
  Int : Integrator  ExternalReset=falling
  Rel1 : Relay  OnSwitchValue=DT  OutDataType=sfix(16)  OutScaling=2^0
  s1d : Outport  InitialOutput=0
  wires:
  Rel1/1 -> s1d/1
  s1/1 -> Int/1, Int/2
  Int/1 -> Rel1/1

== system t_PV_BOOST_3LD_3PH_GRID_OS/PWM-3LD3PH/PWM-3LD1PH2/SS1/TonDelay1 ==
  s1 : Inport  Orientation=down  OutDataType=sfix(16)  OutScaling=2^0
  Int : Integrator  ExternalReset=falling
  Rel1 : Relay  OnSwitchValue=DT  OutDataType=sfix(16)  OutScaling=2^0
  s1d : Outport  InitialOutput=0
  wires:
  Rel1/1 -> s1d/1
  s1/1 -> Int/1, Int/2
  Int/1 -> Rel1/1

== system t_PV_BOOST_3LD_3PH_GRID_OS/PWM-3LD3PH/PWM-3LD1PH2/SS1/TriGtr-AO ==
  Ampl. : Gain  Gain=A  ParameterDataType=sfix(16)  ParameterScaling=2^0  OutDataType=sfix(16)  OutScaling=2^0
  Offset : Constant  Value=O  OutDataType=sfix(16)  OutScaling=2^0
  Sum : Sum  OutDataType=sfix(16)  OutScaling=2^0
  TriGtr1 : Subsystem  mask(TriGtr){T=T, Td=Td}
      mask prompts: T "Period Time"; Td "Time Delay"
      mask help: Triangular Wave Generator with variable time delay
  Out1 : Outport
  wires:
  Offset/1 -> Sum/2
  TriGtr1/1(O) -> Ampl./1
  Ampl./1 -> Sum/1
  Sum/1 -> Out1/1

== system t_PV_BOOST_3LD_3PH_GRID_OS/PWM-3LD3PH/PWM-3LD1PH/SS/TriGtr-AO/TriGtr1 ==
  Clock : Clock
  S2 : Subsystem
  Sum : Sum  OutDataType=sfix(16)  OutScaling=2^0
  T : Constant  Value=T  OutDataType=sfix(16)  OutScaling=2^0
  Td : Constant  Value=Td  OutDataType=sfix(16)  OutScaling=2^0
  mod : Math  Operator=mod
  O : Outport  InitialOutput=0
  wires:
  Td/1 -> Sum/2
  Sum/1 -> mod/1
  T/1 -> mod/2
  Clock/1 -> Sum/1
  S2/1(O1) -> O/1
  mod/1 -> S2/1(I1)

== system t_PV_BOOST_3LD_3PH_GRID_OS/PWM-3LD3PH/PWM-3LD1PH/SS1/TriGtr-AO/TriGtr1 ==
  Clock : Clock
  S1 : Subsystem
  Sum : Sum
  T : Constant  Value=T
  Td : Constant  Value=Td
  mod : Math  Operator=mod
  O : Outport  InitialOutput=0
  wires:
  Td/1 -> Sum/2
  Sum/1 -> mod/1
  T/1 -> mod/2
  Clock/1 -> Sum/1
  S1/1(O1) -> O/1
  mod/1 -> S1/1(I1)

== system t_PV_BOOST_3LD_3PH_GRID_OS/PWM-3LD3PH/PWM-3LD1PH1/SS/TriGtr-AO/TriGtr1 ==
  Clock : Clock
  S2 : Subsystem
  Sum : Sum  OutDataType=sfix(16)  OutScaling=2^0
  T : Constant  Value=T  OutDataType=sfix(16)  OutScaling=2^0
  Td : Constant  Value=Td  OutDataType=sfix(16)  OutScaling=2^0
  mod : Math  Operator=mod
  O : Outport  InitialOutput=0
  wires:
  mod/1 -> S2/1(I1)
  S2/1(O1) -> O/1
  Clock/1 -> Sum/1
  T/1 -> mod/2
  Sum/1 -> mod/1
  Td/1 -> Sum/2

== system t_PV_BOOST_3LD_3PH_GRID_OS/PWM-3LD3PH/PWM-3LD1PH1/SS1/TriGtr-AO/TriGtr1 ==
  Clock : Clock
  S1 : Subsystem
  Sum : Sum
  T : Constant  Value=T
  Td : Constant  Value=Td
  mod : Math  Operator=mod
  O : Outport  InitialOutput=0
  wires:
  mod/1 -> S1/1(I1)
  S1/1(O1) -> O/1
  Clock/1 -> Sum/1
  T/1 -> mod/2
  Sum/1 -> mod/1
  Td/1 -> Sum/2

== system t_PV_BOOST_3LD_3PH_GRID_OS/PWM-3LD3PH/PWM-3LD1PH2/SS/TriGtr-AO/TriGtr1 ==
  Clock : Clock
  S2 : Subsystem
  Sum : Sum  OutDataType=sfix(16)  OutScaling=2^0
  T : Constant  Value=T  OutDataType=sfix(16)  OutScaling=2^0
  Td : Constant  Value=Td  OutDataType=sfix(16)  OutScaling=2^0
  mod : Math  Operator=mod
  O : Outport  InitialOutput=0
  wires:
  Td/1 -> Sum/2
  Sum/1 -> mod/1
  T/1 -> mod/2
  Clock/1 -> Sum/1
  S2/1(O1) -> O/1
  mod/1 -> S2/1(I1)

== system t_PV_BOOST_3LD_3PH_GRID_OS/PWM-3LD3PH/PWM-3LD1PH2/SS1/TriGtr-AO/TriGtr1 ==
  Clock : Clock
  S1 : Subsystem
  Sum : Sum
  T : Constant  Value=T
  Td : Constant  Value=Td
  mod : Math  Operator=mod
  O : Outport  InitialOutput=0
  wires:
  Td/1 -> Sum/2
  Sum/1 -> mod/1
  T/1 -> mod/2
  Clock/1 -> Sum/1
  S1/1(O1) -> O/1
  mod/1 -> S1/1(I1)

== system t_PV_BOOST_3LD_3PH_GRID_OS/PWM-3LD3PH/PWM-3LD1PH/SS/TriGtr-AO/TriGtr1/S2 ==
  I1 : Inport
  Fcn : Fcn  Expr="(u* (u <=T/4) * 4/T)   +  (  (u > T/4) && ( u <=3*T/4) )* ( 1 - (u-T/4) *4/T )   +  ( (u > 3*T/4)&& (u<=T)) * ( ((u -3*T/4)* 4/T )-1 )"
  O1 : Outport
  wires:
  Fcn/1 -> O1/1
  I1/1 -> Fcn/1

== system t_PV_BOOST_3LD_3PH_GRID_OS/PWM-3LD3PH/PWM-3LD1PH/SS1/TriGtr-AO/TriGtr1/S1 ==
  I1 : Inport
  Fcn : Fcn  Expr="(u* (u <=T/4) * 4/T)   +  (  (u > T/4) && ( u <=3*T/4) )* ( 1 - (u-T/4) *4/T )   +  ( (u > 3*T/4)&& (u<=T)) * ( ((u -3*T/4)* 4/T )-1 )"
  O1 : Outport
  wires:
  I1/1 -> Fcn/1
  Fcn/1 -> O1/1

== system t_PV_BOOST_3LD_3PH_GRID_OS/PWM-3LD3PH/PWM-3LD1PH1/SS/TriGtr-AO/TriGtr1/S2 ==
  I1 : Inport
  Fcn : Fcn  Expr="(u* (u <=T/4) * 4/T)   +  (  (u > T/4) && ( u <=3*T/4) )* ( 1 - (u-T/4) *4/T )   +  ( (u > 3*T/4)&& (u<=T)) * ( ((u -3*T/4)* 4/T )-1 )"
  O1 : Outport
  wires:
  I1/1 -> Fcn/1
  Fcn/1 -> O1/1

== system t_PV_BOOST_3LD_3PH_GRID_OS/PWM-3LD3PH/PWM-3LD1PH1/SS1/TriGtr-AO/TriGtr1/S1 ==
  I1 : Inport
  Fcn : Fcn  Expr="(u* (u <=T/4) * 4/T)   +  (  (u > T/4) && ( u <=3*T/4) )* ( 1 - (u-T/4) *4/T )   +  ( (u > 3*T/4)&& (u<=T)) * ( ((u -3*T/4)* 4/T )-1 )"
  O1 : Outport
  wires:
  Fcn/1 -> O1/1
  I1/1 -> Fcn/1

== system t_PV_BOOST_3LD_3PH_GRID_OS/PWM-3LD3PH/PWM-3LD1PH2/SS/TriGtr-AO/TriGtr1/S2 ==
  I1 : Inport
  Fcn : Fcn  Expr="(u* (u <=T/4) * 4/T)   +  (  (u > T/4) && ( u <=3*T/4) )* ( 1 - (u-T/4) *4/T )   +  ( (u > 3*T/4)&& (u<=T)) * ( ((u -3*T/4)* 4/T )-1 )"
  O1 : Outport
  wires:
  Fcn/1 -> O1/1
  I1/1 -> Fcn/1

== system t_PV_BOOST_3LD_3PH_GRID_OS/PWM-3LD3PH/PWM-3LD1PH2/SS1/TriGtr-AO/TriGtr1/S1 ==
  I1 : Inport
  Fcn : Fcn  Expr="(u* (u <=T/4) * 4/T)   +  (  (u > T/4) && ( u <=3*T/4) )* ( 1 - (u-T/4) *4/T )   +  ( (u > 3*T/4)&& (u<=T)) * ( ((u -3*T/4)* 4/T )-1 )"
  O1 : Outport
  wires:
  I1/1 -> Fcn/1
  Fcn/1 -> O1/1
